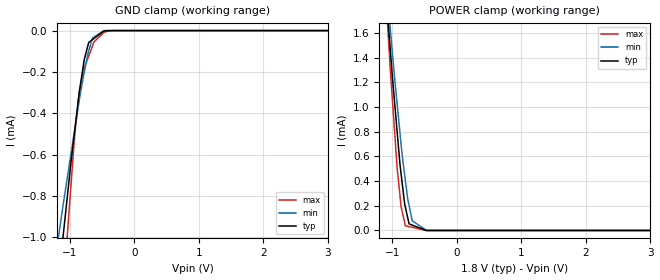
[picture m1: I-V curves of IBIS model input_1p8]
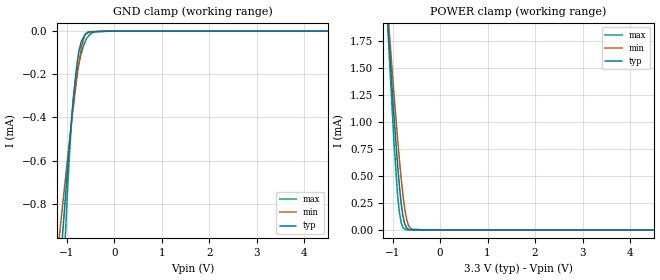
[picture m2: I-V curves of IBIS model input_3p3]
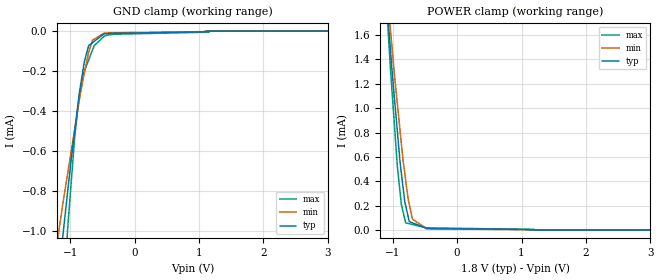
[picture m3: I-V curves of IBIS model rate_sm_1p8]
|Texas Instruments Incorporated
| 112dB SNR Low-Power Mono Audio ADC
| Marketing part#   Digital Voltage Range   Package-type   #pins
| PCM4201PW   1.65V-3.6V   TSSOP   16
| PCM4201PWG4   1.65V-3.6V   TSSOP   16
| PCM4201PWR   1.65V-3.6V   TSSOP   16
| PCM4201PWRG4   1.65V-3.6V   TSSOP   16
[IBIS Ver]   3.2
[File name]   pcm4201.ibs
|SIMDE Ver   V3.0 - 201101 - RHL4 - Build 457
[File Rev]   1.0
[Date]   6/15/2011
[Source]
| Texas Instruments Incorporated.
| Analog-eLab Design Center, HPA
| 12500 TI Blvd
| Dallas, TX -75243
| e-mail: elab_ibis@list.ti.com
[Notes]   Revision History:
| Rev 1.0: 6/15/2011
| - Initial version of the model
| - Model generated from simulations in TISPICE
| - Model matched to SPICE simulation
| - C_comp although listed in numerical order of value are
|   obtained from varying PVT conditions. For PVT conditions for
|   each specific value refer the buffer description under
|   respective [Model]. IBIS model user is responsible for using
|   appropriate C_comp to simulate for Signal Integrity.
| - Model names with a trailing _1p8 contains the model for
|   1.8V [1.71V and 1.89V].Model names with a trailing _3p3
|   contains the model for 3.3V [3.0V and 3.6V].
|*   EXCEPTION:   *
|*   - For model RATE_SM there will be a leakage current in the   *
|*   clamp I-V table because of the pulldown/pullup on pad.   *
[Disclaimer]
| This model is designed as an aid for customers of Texas Instruments.
| TI and its licensors and suppliers make no warranties, either expressed
| or implied, with respect to this  model, including the warranties of
| merchantability or fitness for a particular purpose. The model is
| provided solely on an "as is" basis. The entire risk as to its quality
| and performance is with the customer.
[Copyright]
 (C) Copyright 2011 Texas Instruments Incorporated.All rights reserved.
|   PCM4201
[Component]   PCM4201
[Manufacturer]   TI
[Package]   |16 TSSOP  -  PW package
|   typ   min   max
R_pkg   0.14914   0.08461   0.19020
L_pkg   2.18361nH   1.69526nH   2.83570nH
C_pkg   0.28057pF   0.24147pF   0.35977pF
[Pin]  signal_name   model_name   R_pin   L_pin   C_pin
1   VIN+   TERM   0.16106   2.82913nH  0.33451pF
2   VIN-   TERM   0.17262   2.06207nH  0.25787pF
3   AGND   GND   0.04517   1.32608nH  0.28544pF
4   VCC   POWER   0.04514   1.32000nH  0.28424pF
5   RATE   RATE_SM   0.12892   1.69526nH  0.24161pF
6   S/_M   RATE_SM   0.12911   1.69737nH  0.24199pF
7   _RST   INPUT   0.17037   2.04532nH  0.25600pF
8   HPFD   INPUT   0.16109   2.83570nH  0.33546pF
9   DATA   DATA   0.16106   2.83540nH  0.33549pF
10   FSYNC   SYNC_BCK   0.17262   2.06432nH  0.25676pF
11   BCK   SYNC_BCK   0.12911   1.69737nH  0.24196pF
12   SCKI   INPUT   0.12892   1.69526nH  0.24147pF
13   VDD   POWER   0.06672   1.44032nH  0.26341pF
14   DGND   GND   0.04533   1.32967nH  0.28301pF
15   VREF-   TERM   0.19020   2.21147nH  0.26397pF
16   VREF+   TERM   0.08461   2.53469nH  0.35977pF
|   Model Selectors
[Model Selector] INPUT
input_1p8   1.8V digital input
input_3p3   3.3V digital input
[Model Selector] RATE_SM
rate_sm_1p8   1.8V digital input
rate_sm_3p3   3.3V digital input
[Model Selector] DATA
data_ds_1p8   1.8V double-speed digital output
data_ds_3p3   3.3V double-speed digital output
data_lp_1p8   1.8V low-power digital output
data_lp_3p3   3.3V low-power digital output
[Model Selector] SYNC_BCK
sycbck_ds_1p8   1.8V double-speed digital I/O
sycbck_ds_3p3   3.3V double-speed digital I/O
sycbck_lp_1p8   1.8V low-power digital I/O
sycbck_lp_3p3   3.3V low-power digital I/O
[Model Selector] TERM
term_1-8V   1.8V nominal termination
term_3-3V   3.3V nominal termination
[Model] term_1-8V
Model_type Terminator
C_comp   1.0e-20F  1.0e-20F  1.0e-20F
|   typ   min   max
[Voltage Range]   1.8V   1.71V   1.89V
[POWER Clamp Reference]   1.8V   1.71V   1.89V
[GND Clamp Reference]   0V   0V   0V
|Ambient Temperature   25   70   -10
|Junction Temperature
[Temperature Range]   35   80   -10
[Model] term_3-3V
Model_type Terminator
C_comp   1.0e-20F  1.0e-20F  1.0e-20F
|   typ   min   max
[Voltage Range]   3.3V   3.0V   3.6V
[POWER Clamp Reference]   3.3V   3.0V   3.6V
[GND Clamp Reference]   0V   0V   0V
|Ambient Temperature   25   70   -10
|Junction Temperature
[Temperature Range]   35   80   -10
| Models and submodels in the file (14): input_1p8 (Input), input_3p3 (Input), rate_sm_1p8 (Input), rate_sm_3p3 (Input), data_ds_1p8 (Output), data_ds_3p3 (Output), data_lp_1p8 (Output), data_lp_3p3 (Output), sycbck_ds_1p8 (I/O), sycbck_ds_3p3 (I/O), sycbck_lp_1p8 (I/O), sycbck_lp_3p3 (I/O), term_1-8V (Terminator), term_3-3V (Terminator)
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|   input_1p8 Model
[Model]   input_1p8
Model_type   Input
Vinl = 0.54
Vinh = 1.26
|   typ   min   max
|   (nom PVT)   (fast PVT)   (slow PVT)
|C_comp from frequency sweep method (F=27.65MHz)
|Average
|C_comp   9.432e-13   8.111e-13   1.080e-12
|C_comp from LC tank measurement(L=1nH)
|Average
|Resonant Frequency(Hz)   8.761e+10   8.791e+10   2.620e+10
C_comp   3.303e-15   3.281e-15   3.694e-14
| Where nom  PVT is Nominal Process, 1.8V, 35C
|   Fast PVT is Strong Process,  1.89V, -10C
|   Slow PVT is Weak Process,   1.71V, 80C
[Model Spec]
Vinl   0.54   0.513   0.567
Vinh   1.26   1.197   1.323
[Voltage Range]   1.8   1.71   1.89
|Ambient Temperature   25   70   -10
|Junction Temperature
[Temperature Range]   35   80   -10
[Power Clamp Reference]   1.8   1.71   1.89
[GND Clamp Reference]   0   0   0
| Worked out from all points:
|   GND clamp passes 1 mA (typ) near -1.11 V on its own axis
|   POWER clamp passes 1 mA (typ) near -0.96 V on its own axis
[GND Clamp]
|   Voltage   I(typ)   I(min)   I(max)
-1.8V     -3.16mA    -2.36mA    -4.894mA
-1.165V   -1.174mA   -975uA     -1.599mA
-1.115V   -1.028mA   -866.7uA   -1.358mA
-1.04V    -806.2uA   -713.7uA   -992uA
-981mV    -634.2uA   -595uA     -743.8uA
-926.1mV  -489.4uA   -483.7uA   -513.1uA
-856.2mV  -304.9uA   -341.8uA   -306uA
-775.8mV  -139.5uA   -200.5uA   -181.5uA
-707.4mV  -57.71uA   -97.54uA   -123.2uA
-648.1mV  -43.59uA   -35.62uA   -73.63uA
-470.3mV  -1.537uA   -423.8nA   -8.455uA
3.6V      0A         0A         0A
[POWER Clamp]
|   Voltage   I(typ)   I(min)   I(max)
-1.8V     7.028mA    6.466mA    8.447mA
-1.141V   2.209mA    2.277mA    2.26mA
-1.032V   1.467mA    1.634mA    1.309mA
-922.3mV  783.6uA    1.01mA     489.5uA
-882mV    541.2uA    793.7uA    286.9uA
-861.8mV  449.3uA    685.6uA    185.6uA
-797.6mV  187.9uA    404uA      38.18uA
-761mV    102.4uA    253.4uA    33.9uA
-739.8mV  52.99uA    200.8uA    31.43uA
-690.8mV  43.32uA    79uA       25.71uA
-470.3mV  16.69nA    280.2nA    0A
3.6V      0A         0A         0A
|   input_3p3 Model
[Model]   input_3p3
Model_type   Input
Vinl = 0.99
Vinh = 2.31
|   typ   min   max
|   (nom PVT)   (fast PVT)   (slow PVT)
|C_comp from frequency sweep method (F=27.65MHz)
|Average
|C_comp   8.075e-13   6.905e-13   9.388e-13
|C_comp from LC tank measurement(L=1nH)
|Average
|Resonant Frequency(Hz)   8.761e+10   8.761e+10   2.892e+10
C_comp   3.303e-15   3.303e-15   3.032e-14
| Where nom  PVT is Nominal Process, 3.3V, 35C
|   Fast PVT is Strong Process,  3.6V, -10C
|   Slow PVT is Weak Process,   3V, 80C
[Model Spec]
Vinl   0.99   0.9   1.08
Vinh   2.31   2.1   2.52
[Voltage Range]   3.3   3   3.6
|Ambient Temperature   25   70   -10
|Junction Temperature
[Temperature Range]   35   80   -10
[Power Clamp Reference]   3.3   3   3.6
[GND Clamp Reference]   0   0   0
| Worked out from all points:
|   GND clamp passes 1 mA (typ) near -1.11 V on its own axis
|   POWER clamp passes 1 mA (typ) near -0.96 V on its own axis
[GND Clamp]
|   Voltage   I(typ)   I(min)   I(max)
-3.3V     -7.983mA   -5.734mA   -12.93mA
-1.145V   -1.116mA   -931.3uA   -1.499mA
-1.08V    -923.9uA   -793.6uA   -1.183mA
-1.003V   -697.8uA   -634.7uA   -834.3uA
-896.4mV  -405.5uA   -419.5uA   -413.8uA
-860.4mV  -316.4uA   -353.3uA   -316.6uA
-778.8mV  -145.3uA   -203.7uA   -185.9uA
-693mV    -48.13uA   -78.49uA   -103.3uA
-627mV    -20.04uA   -22.93uA   -57.81uA
-546mV    -6.981uA   -3.091uA   -24.41uA
-133.2mV  -952.5nA   0A         0A
6.6V      0A         0A         0A
[POWER Clamp]
|   Voltage   I(typ)   I(min)   I(max)
-3.3V     18.4mA     16.38mA    23.05mA
-1.129V   2.119mA    2.206mA    2.151mA
-1.076V   1.767mA    1.89mA     1.686mA
-972mV    1.079mA    1.279mA    835.8uA
-896.4mV  621.2uA    864.4uA    341.7uA
-856.8mV  416.7uA    663.8uA    168.7uA
-817.2mV  246.3uA    478.9uA    66.53uA
-782.1mV  134.9uA    332.9uA    26.88uA
-705.6mV  22.4uA     106.9uA    1.693uA
-591mV    3.449uA    7.184uA    272.8nA
-285mV    1.653uA    0A         0A
6.6V      0A         0A         0A
|   rate_sm_1p8 Model
[Model]   rate_sm_1p8
Model_type   Input
Vinl = 0.54
Vinh = 1.26
|   typ   min   max
|   (nom PVT)   (fast PVT)   (slow PVT)
|C_comp from frequency sweep method (F=27.65MHz)
|Average
|C_comp   1.080e-12   9.538e-13   1.215e-12
|C_comp from LC tank measurement(L=1nH)
|Average
|Resonant Frequency(Hz)   9.344e+10   9.568e+10   8.319e+10
C_comp   2.904e-15   2.770e-15   3.664e-15
| Where nom  PVT is Nominal Process, 1.8V, 35C
|   Fast PVT is Strong Process,  1.89V, -10C
|   Slow PVT is Weak Process,   1.71V, 80C
[Model Spec]
Vinl   0.54   0.513   0.567
Vinh   1.26   1.197   1.323
[Voltage Range]   1.8   1.71   1.89
|Ambient Temperature   25   70   -10
|Junction Temperature
[Temperature Range]   35   80   -10
[Power Clamp Reference]   1.8   1.71   1.89
[GND Clamp Reference]   0   0   0
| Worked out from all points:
|   GND clamp passes 1 mA (typ) near -1.10 V on its own axis
|   POWER clamp passes 1 mA (typ) near -0.96 V on its own axis
[GND Clamp]
|   Voltage   I(typ)   I(min)   I(max)
-1.8V     -3.16mA    -2.361mA   -4.895mA
-1.168V   -1.186mA   -983.6uA   -1.619mA
-1.115V   -1.029mA   -867.5uA   -1.361mA
-1.04V    -807.8uA   -714.9uA   -995.5uA
-931.8mV  -507.4uA   -496.8uA   -541.2uA
-859.9mV  -318.2uA   -351.5uA   -327.4uA
-779.4mV  -153uA     -209.7uA   -203.2uA
-711mV    -71.78uA   -106.5uA   -143.4uA
-651.5mV  -57.45uA   -45.41uA   -93.57uA
-470.3mV  -14.06uA   -9.9uA     -25.67uA
1.162V    0A         0A         0A
3.6V      0A         0A         0A
[POWER Clamp]
|   Voltage   I(typ)   I(min)   I(max)
-1.8V     7.028mA    6.467mA    8.447mA
-1.142V   2.223mA    2.289mA    2.277mA
-1.034V   1.482mA    1.647mA    1.329mA
-924.2mV  799uA      1.026mA    511.1uA
-863.7mV  465.2uA    706.9uA    209.1uA
-810mV    229.2uA    460.5uA    86.69uA
-797.6mV  200.1uA    409.8uA    58.38uA
-761mV    114.3uA    260.1uA    53.75uA
-741.6mV  68.94uA    212.7uA    51.3uA
-690.8mV  58.32uA    88.3uA     44.89uA
-470.3mV  12.45uA    9.742uA    17.03uA
3.6V      0A         0A         0A
